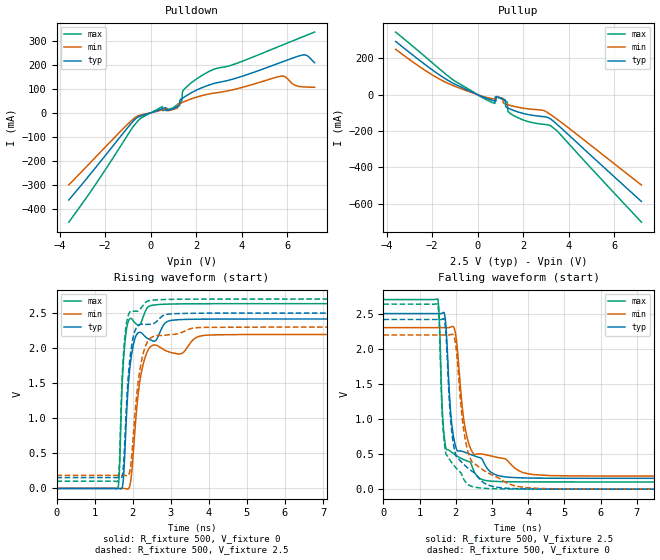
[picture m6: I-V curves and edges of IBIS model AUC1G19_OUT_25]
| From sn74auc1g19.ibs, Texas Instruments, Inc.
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[Model]   AUC1G19_OUT_25
Model_type  Output
Vref =   0
Rref =   500
Cref =   30p
Vmeas =   1.25
| variable   typ   min   max
C_comp   8.42pF   0.47pF   23.62pF
| C_pullup   8.42pF   0.47pF   23.62pF
| C_pulldown   8.42pF   0.47pF   23.62pF
[Temperature Range]   40   100   -40
| Ambient temperature   25   85   -40
[Voltage range]   2.5   2.3   2.7
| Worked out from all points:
|   slope of the pulldown table from 0 to 0.375 V, typ, clamps not added: 30.9 ohm
|   slope of the pullup table from 0 to 0.375 V, typ, clamps not added: 19.2 ohm
|   rising waveform, R_fixture 500, V_fixture 0: 20-80 % time 187ps typ, 263ps min, 133ps max; typ from 0 V to 2.42 V
|   falling waveform, R_fixture 500, V_fixture 2.5: 20-80 % time 228ps typ, 322ps min, 152ps max; typ from 2.5 V to 0.154 V
|   rising waveform, R_fixture 500, V_fixture 2.5: 20-80 % time 184ps typ, 260ps min, 131ps max; typ from 0.154 V to 2.5 V
|   falling waveform, R_fixture 500, V_fixture 0: 20-80 % time 243ps typ, 346ps min, 156ps max; typ from 2.42 V to 0 V
[Pulldown]
| AUC1G19_OUT_25
|   Voltage   I(typ)   I(min)   I(max)
-3.6V     -361.7mA   -299.1mA   -453.9mA
-445mV    -13.39mA   -9.087mA   -23.05mA
515mV     17.02mA    12.57mA    25.99mA
1.03V     19.08mA    15.52mA    23.89mA
1.27V     30.04mA    38.39mA    41.38mA
1.37V     59.36mA    42.45mA    48.97mA
1.395V    60.88mA    43.46mA    85.17mA
1.48V     65.99mA    46.82mA    98.83mA
2.545V    114.9mA    77.95mA    170.8mA
5.71V     209mA      152mA      278.4mA
6.745V    240.7mA    107.5mA    318mA
7.2V      207.8mA    106.1mA    335.1mA
[Pullup]
| AUC1G19_OUT_25
|   Voltage   I(typ)   I(min)   I(max)
-3.6V     292.7mA    249.8mA    344.4mA
-960mV    55.5mA     44.14mA    71.53mA
730mV     -33.82mA   -24.42mA   -47.21mA
760mV     -34.84mA   -25.13mA   -47.16mA
770mV     -35.18mA   -25.36mA   -13.07mA
1.115V    -23.84mA   -20.26mA   -27.67mA
1.215V    -28.81mA   -50.48mA   -34.67mA
1.295V    -71.05mA   -53.78mA   -40.2mA
1.345V    -74.3mA    -55.73mA   -93.3mA
1.755V    -94.43mA   -68.81mA   -126mA
3.305V    -143.2mA   -118.1mA   -180.1mA
7.2V      -588mA     -497.7mA   -701.8mA
[Ramp]
| AUC1G19_OUT_25
| variable   typ   min   max
dV/dt_r   1.45/1.88E-10   1.32/2.64E-10   1.59/1.34E-10
dV/dt_f   1.42/2.27E-10   1.28/3.23E-10   1.56/1.53E-10
R_load = 500
[Rising Waveform]
| AUC1G19_OUT_25
R_fixture =   500
C_fixture =   0
L_fixture =   0
V_fixture =   0
V_fixture_min = 0
V_fixture_max = 0
|   Time   V(typ)   V(min)   V(max)
0s        9.76nV     28.57nV    1.856nV
1.61ns    832.4uV    -7.102uV   7.732mV
1.745ns   75.55mV    1.157mV    1.711V
1.85ns    1.166V     -7.282mV   2.307V
1.95ns    1.825V     113.6mV    2.425V
2.07ns    2.154V     905.2mV    2.356V
2.235ns   2.216V     1.673V     2.381V
2.49ns    2.111V     2.031V     2.61V
3.38ns    2.41V      1.969V     2.632V
23ns      2.416V     2.195V     2.634V
[Falling Waveform]
| AUC1G19_OUT_25
R_fixture =   500
C_fixture =   0
L_fixture =   0
V_fixture =   2.5
V_fixture_min = 2.3
V_fixture_max = 2.7
|   Time   V(typ)   V(min)   V(max)
0s        2.5V       2.3V       2.7V
1.505ns   2.5V       2.3V       2.707V
1.63ns    2.506V     2.3V       1.097V
1.725ns   2.337V     2.299V     587.3mV
1.86ns    1.082V     2.308V     536.1mV
2ns       601.5mV    2.189V     482.9mV
2.305ns   515.5mV    753.6mV    403.4mV
2.79ns    364.1mV    493.4mV    127.7mV
4.61ns    155.8mV    193.4mV    103mV
23ns      154.5mV    186.3mV    102.6mV
[Rising Waveform]
| AUC1G19_OUT_25
R_fixture =   500
C_fixture =   0
L_fixture =   0
V_fixture =   2.5
V_fixture_min = 2.3
V_fixture_max = 2.7
|   Time   V(typ)   V(min)   V(max)
0s        154.5mV    186.3mV    102.6mV
1.61ns    155.3mV    186.2mV    111.5mV
1.65ns    153.1mV    186.3mV    351.1mV
1.745ns   243mV      187.3mV    1.802V
1.845ns   1.271V     181.7mV    2.381V
1.94ns    1.902V     293.3mV    2.523V
2.04ns    2.213V     918.8mV    2.527V
2.205ns   2.341V     1.741V     2.562V
2.43ns    2.34V      2.122V     2.678V
23ns      2.5V       2.3V       2.7V
[Falling Waveform]
| AUC1G19_OUT_25
R_fixture =   500
C_fixture =   0
L_fixture =   0
V_fixture =   0
V_fixture_min = 0
V_fixture_max = 0
|   Time   V(typ)   V(min)   V(max)
0s        2.416V     2.195V     2.634V
1.505ns   2.416V     2.195V     2.638V
1.63ns    2.42V      2.195V     1.016V
1.715ns   2.291V     2.195V     530.3mV
1.845ns   1.068V     2.199V     409.8mV
1.955ns   584.5mV    2.167V     332.4mV
2.23ns    348.5mV    806.2mV    132.8mV
2.5ns     238.7mV    368.2mV    30.71mV
4.375ns   1.753mV    9.096mV    400.2uV
23ns      18.88uV    1.595uV    8.905uV
